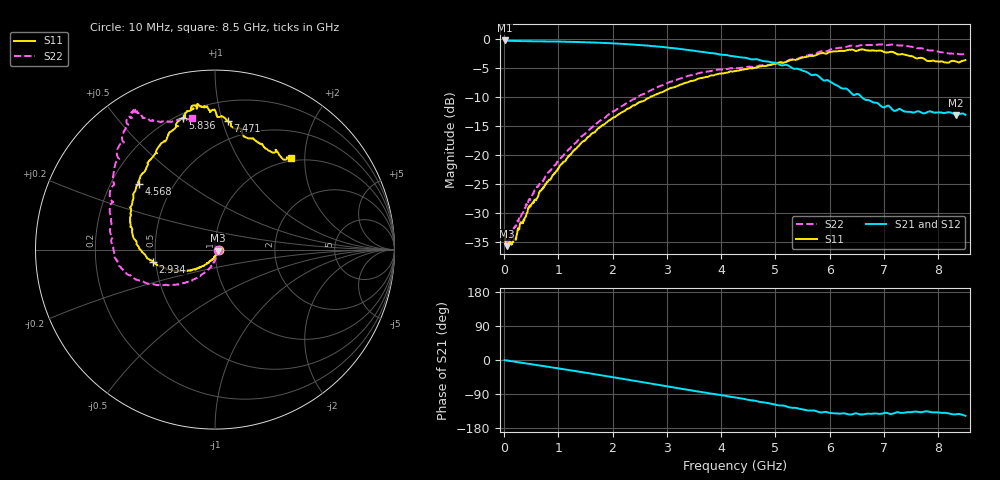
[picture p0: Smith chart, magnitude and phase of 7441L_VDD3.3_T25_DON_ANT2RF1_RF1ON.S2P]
!Agilent Technologies,E5071C,MY46417908,A.11.23
!Date: Mon May 03 19:53:33 2021
!Data & Calibration Information:
!Freq	S11:SOLT2(ON)	S21:SOLT2(ON)	S12:SOLT2(ON)	S22:SOLT2(ON)
!PortZ  Port1:50+j0  Port2:50+j0
!Above PortZ is port z conversion or system Z0 setting when saving the data.
!When reading, reference impedance value at option line is always used.
# Hz S dB R 50
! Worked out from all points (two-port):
!   1601 points, 10 MHz to 8.5 GHz, reference 50 ohm
!   highest |S21| = -0.21 dB at 10 MHz (marker M1); lowest = -13.1 dB at 8.33 GHz (marker M2)
!   |S21| within 3 dB of the highest: start of sweep to 4.462 GHz
!   lowest |S11| = -35.8 dB at 52.45 MHz (marker M3), VSWR 1.03, Z = 51.6 - j0.53 ohm
!   |S11| at or under -10 dB: start of sweep to 2.69 GHz
!   |S22| runs from -35.4 to -0.9 dB; largest |S21 - S12| = 0.0098
!   S11 on the Smith chart (normalised r, x): 10 MHz: 1.04, -0.00; 2.934 GHz: 0.48, -0.07; 4.568 GHz: 0.32, +0.34; 5.836 GHz: 0.22, +0.76; 7.471 GHz: 0.35, +1.04; 8.5 GHz: 0.95, +1.71
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1e7  -33.80 -1.3  -0.21 -0.4  -0.21 -0.4  -34.80 -12.0
5.245e7  -35.76 -18.4  -0.26 -1.3  -0.26 -1.3  -34.86 -22.0
1.851062e8  -34.62 -50.5  -0.29 -4.3  -0.30 -4.3  -32.57 -47.8
4.610312e8  -29.05 -83.8  -0.34 -10.3  -0.34 -10.3  -27.65 -79.0
5.883812e8  -27.82 -93.1  -0.35 -13.1  -0.35 -13.0  -25.79 -86.1
1.050025e9  -21.59 -116.3  -0.41 -23.3  -0.42 -23.3  -20.50 -102.3
1.426769e9  -17.88 -129.4  -0.50 -31.8  -0.50 -31.8  -16.82 -115.3
2.185562e9  -12.56 -149.0  -0.80 -49.7  -0.81 -49.7  -11.48 -134.8
2.843538e9  -9.38 -166.3  -1.28 -65.6  -1.29 -65.7  -8.20 -150.1
2.933744e9  -9.08 -169.1  -1.34 -67.8  -1.36 -67.9  -7.91 -151.7
3.602331e9  -6.77 171.7  -2.13 -83.8  -2.13 -84.1  -5.82 -165.0
4.255e9  -5.50 150.3  -2.98 -98.9  -2.95 -99.4  -5.00 -178.1
4.568069e9  -5.03 139.5  -3.48 -106.2  -3.42 -106.5  -4.81 173.5
5.241962e9  -3.72 119.0  -4.57 -124.5  -4.57 -124.7  -3.62 152.9
5.671769e9  -2.87 106.7  -6.19 -133.1  -6.19 -133.6  -2.67 137.0
5.836262e9  -2.44 103.8  -6.73 -138.3  -6.76 -138.8  -2.09 132.9
6.404031e9  -1.80 97.1  -9.37 -143.5  -9.41 -144.3  -1.09 123.2
7.088538e9  -2.23 91.8  -11.50 -141.4  -11.43 -142.0  -0.98 120.6
7.470588e9  -2.86 84.3  -12.53 -137.7  -12.52 -137.6  -1.24 119.2
7.916312e9  -3.72 70.6  -12.66 -138.1  -12.72 -138.1  -1.99 115.4
8.3302e9  -3.83 56.7  -13.09 -143.0  -13.11 -143.4  -2.49 105.0
8.5e9  -3.60 50.4  -13.06 -147.3  -13.08 -147.3  -2.56 100.0
